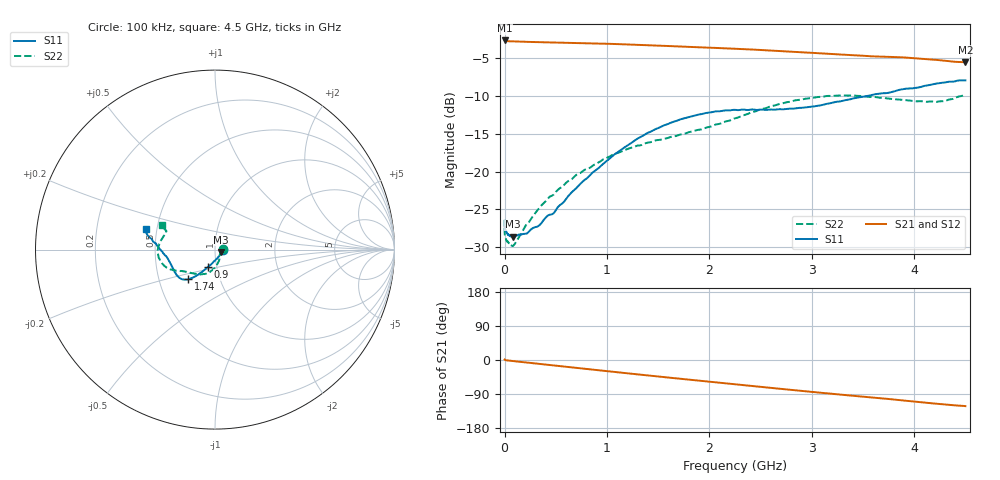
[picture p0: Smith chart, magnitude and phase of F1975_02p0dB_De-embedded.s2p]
! Integrated Device Technology
! Corporate Headquarters
! 6024 Silver Creek Valley Road
! San Jose, CA 95138  USA
! Phone:  1-408-284-8200
! Toll Free:  1-800-223-1366
! Webpage:  http://www.idt.com/
! Timing and RF Division
! 515 Groton Road, Suite 102
! Westford, MA 01886-6024
! Device:  F1975
! Description: 6-bit, 75 ohm, 0.5 dB Digital Step Attenuator
! Frequency:  5.0 MHz -  3.00 GHz
! Package:  4x4 mm QFN Plastic Package: 20 pin
! Ports:  2 RF, 11 DC
!  Pin  1  = D5 (16 dB)
!  Pin  2  = RF1  =  Port 1
!  Pin  3  = Serial Data In (DATA)
!  Pin  4  = Serial Clock (CLK)
!  Pin  5  = Serial Latch Enable (LE)
!  Pin  6  = VDD
!  Pin  7  = NC
!  Pin  8  = NC
!  Pin  9  = NC
!  Pin 10  = GND
!  Pin 11  = GND
!  Pin 12  = NC
!  Pin 13  = VMODE
!  Pin 14  = RF2  =  Port 2
!  Pin 15  = D4 (8 dB)
!  Pin 16  = D3 (4 dB)
!  Pin 17  = D2 (2 dB)
!  Pin 18  = NC
!  Pin 19  = D1 (1 dB)
!  Pin 20  = D0 (0.5 dB)
! State:  4
! Atten State:  2.0 dB
! Voltage:  +3.30 Volts
! Current:  0.594 mA
! Data:  The device was measured on a F1975 evaluation board which has
!  individual transmission lines to the RF pins.  Data was collected
!  using a calibrated network analyzer.  The evaluation board was
!  de-embedded using Automatic Fixture Removal (AFR).
!  The reference plane is the edge of the package pin.
! Misc:
!  Action Tracker AT0415
! Date Measured:  2018-02-08
! Date:  2018-03-26  MJV
! Note:
!  Integrated Device Technology supplies this data as a sample of measured
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# GHz S dB R 75
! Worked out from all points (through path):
!   291 points, 100 kHz to 4.5 GHz, reference 75 ohm
!   highest |S21| = -2.64 dB at 100 kHz (marker M1); lowest = -5.5 dB at 4.5 GHz (marker M2)
!   group delay of S21, straight-line fit = 76.2 ps
!   lowest |S11| = -28.6 dB at 80 MHz (marker M3), VSWR 1.08, Z = 80.3 - j2.19 ohm
!   |S11| at or under -10 dB: start of sweep to 3.535 GHz
!   |S22| runs from -29.9 to -9.8 dB; largest |S21 - S12| = 0.00023
!   S11 on the Smith chart (normalised r, x): 100 kHz: 1.10, +0.00; 900 MHz: 0.91, -0.18; 1.74 GHz: 0.70, -0.25; 4.5 GHz: 0.43, +0.12
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0.0001  -26.52 0.1  -2.64 1.2  -2.64 1.2  -27.50 0.9
0.0008  -27.18 -2.1  -2.68 1.0  -2.68 1.0  -28.12 -1.0
0.002  -27.42 -1.9  -2.69 0.8  -2.69 0.8  -28.41 -1.2
0.02  -28.08 -7.3  -2.73 -0.9  -2.73 -0.9  -29.17 -9.1
0.08  -28.62 -21.5  -2.78 -2.7  -2.78 -2.7  -29.88 -25.4
0.22  -28.19 -46.2  -2.83 -6.9  -2.83 -6.9  -26.85 -52.6
0.36  -26.81 -68.0  -2.87 -10.9  -2.87 -10.9  -24.47 -65.8
0.42  -25.84 -74.3  -2.89 -12.7  -2.89 -12.7  -23.62 -70.0
0.48  -25.52 -81.9  -2.91 -14.4  -2.91 -14.4  -23.05 -74.3
0.62  -23.28 -96.7  -2.95 -18.4  -2.95 -18.4  -21.27 -82.5
0.76  -21.36 -104.9  -2.99 -22.5  -2.99 -22.5  -19.99 -89.8
0.9  -19.74 -111.4  -3.04 -26.5  -3.04 -26.5  -18.93 -96.6
1.28  -15.80 -123.2  -3.21 -37.4  -3.21 -37.4  -16.65 -112.7
1.52  -14.12 -128.0  -3.33 -44.1  -3.33 -44.1  -15.79 -121.9
1.74  -13.00 -132.3  -3.46 -50.2  -3.46 -50.2  -15.03 -130.8
2.26  -11.84 -145.1  -3.74 -64.3  -3.74 -64.3  -12.91 -148.0
2.68  -11.74 -159.5  -4.03 -75.7  -4.03 -75.7  -11.07 -157.7
3.02  -11.37 -170.5  -4.29 -84.6  -4.29 -84.6  -10.22 -167.3
3.4  -10.33 -180.0  -4.59 -94.3  -4.59 -94.3  -9.92 179.9
3.76  -9.54 173.8  -4.82 -103.1  -4.82 -103.1  -10.36 169.7
4.22  -8.34 168.3  -5.21 -115.5  -5.21 -115.5  -10.77 159.2
4.5  -7.93 163.1  -5.52 -121.7  -5.52 -121.7  -9.78 155.4
